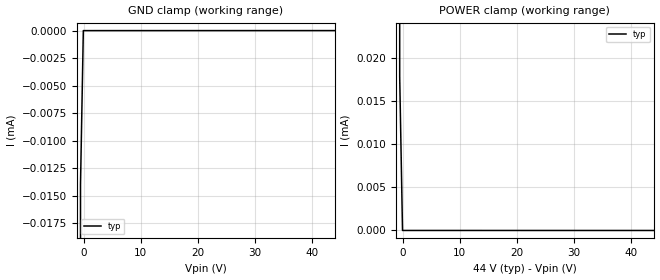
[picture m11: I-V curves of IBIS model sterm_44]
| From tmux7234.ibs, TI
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| sterm_44
[Model]   sterm_44
Model_type   Terminator
|   typ   min   max
C_comp   6.362683e-12   NA   NA
[Voltage Range]   44   NA   NA
[Temperature Range]   27   NA   NA
[Power Clamp Reference]   44   NA   NA
[GND Clamp Reference]   0   NA   NA
[GND Clamp]
|   Voltage   I(typ)   I(min)   I(max)
-5V       -2.158A    NA         NA
-1.04V    -65.21mA   NA         NA
-545.5mV  -13.97uA   NA         NA
-50.51mV  -1.329nA   NA         NA
44V       1.275nA    NA         NA
[POWER Clamp]
|   Voltage   I(typ)   I(min)   I(max)
-5V       2.77A      NA         NA
-1.04V    62.97mA    NA         NA
-545.5mV  17.88uA    NA         NA
-50.5mV   1.281nA    NA         NA
44V       -1.318nA   NA         NA
